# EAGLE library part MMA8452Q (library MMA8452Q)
MMA8452Q 3-Axis, 12/8-bit Digital Accelerometer Supply Voltage: 1.6-3.6V Range: +/- 2g, 4g, 8g Interface: I2C, 12-bit and 8-bit ODR: 1.56 Hz - 800 Hz Package: QFN-16 http://cache.freescale.com/files/sensors/doc/data_sheet/MMA8452Q.pdf
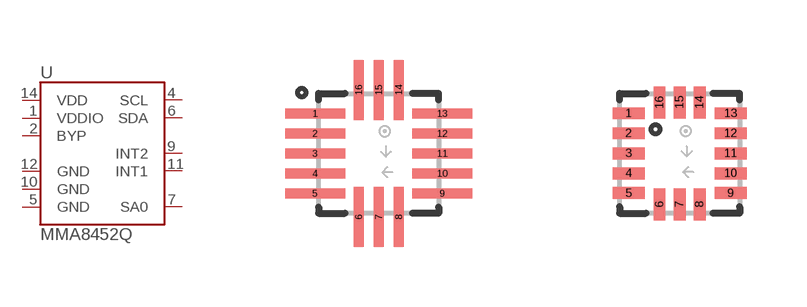
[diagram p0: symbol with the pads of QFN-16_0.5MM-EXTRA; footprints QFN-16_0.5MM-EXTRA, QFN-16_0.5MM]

Designator prefix U

## MMA8452QL (AVAILABILITY: Unavailable; DESCRIPTION: Sensor: accelerometer; Range: 2/4/8g; -40÷85°C; 1.95÷3.6V; MF: NXP Semiconductors; MP: MMA8452Q; PACKAGE: None; PRICE: None)  [QFN-16_0.5MM-EXTRA]
1  VDDIO
2  BYP
4  SCL
5  GND
6  SDA
7  SA0
9  INT2
10  GND
11  INT1
12  GND
14  VDD

## MMA8452QS (AVAILABILITY: Unavailable; DESCRIPTION: Sensor: accelerometer; Range: 2/4/8g; -40÷85°C; 1.95÷3.6V; MF: NXP Semiconductors; MP: MMA8452Q; PACKAGE: None; PRICE: None)  [QFN-16_0.5MM]
Pads as for QFN-16_0.5MM-EXTRA

## Footprint QFN-16_0.5MM-EXTRA (pad centres in mm)
QFN-16 0.5mm Pitch 3 x 3mm Outline 16-pin Used on the MMA8452Q accelerometer Unproven Layout in accordance with App note AN4077 http://cache.freescale.com/files/sensors/doc/app_note/AN4077.pdf
smd 1.5 x 0.25: 1 -1.59,1; 2 -1.59,0.5; 3 -1.59,0; 4 -1.59,-0.5; 5 -1.59,-1; 9 1.59,-1; 10 1.59,-0.5; 11 1.59,0; 12 1.59,0.5; 13 1.59,1
smd 0.25 x 1.5: 6 -0.5,-1.59; 7 0,-1.59; 8 0.5,-1.59; 14 0.5,1.59; 15 0,1.59; 16 -0.5,1.59

## Footprint QFN-16_0.5MM (pad centres in mm)
QFN-16 0.5mm Pitch 3 x 3mm Outline 16-pin Used on the MMA8452Q accelerometer Unproven Layout in accordance with App note AN4077 http://cache.freescale.com/files/sensors/doc/app_note/AN4077.pdf
smd 0.8 x 0.3: 1 -1.275,1; 2 -1.275,0.5; 3 -1.275,0; 4 -1.275,-0.5; 5 -1.275,-1; 9 1.275,-1; 10 1.275,-0.5; 11 1.275,0; 12 1.275,0.5; 13 1.275,1
smd 0.3 x 0.8: 6 -0.5,-1.275; 7 0,-1.275; 8 0.5,-1.275; 14 0.5,1.275; 15 0,1.275; 16 -0.5,1.275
